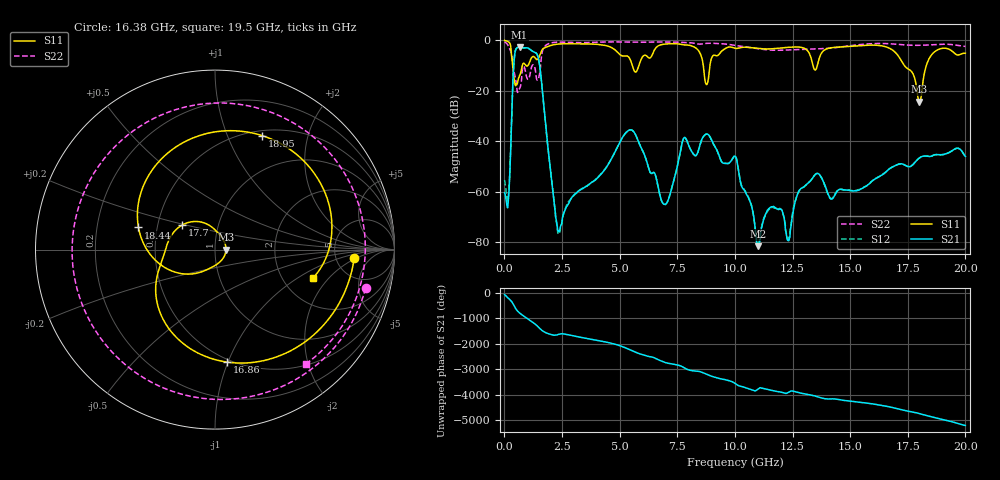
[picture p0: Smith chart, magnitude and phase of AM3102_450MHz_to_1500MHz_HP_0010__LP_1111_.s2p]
!Agilent Technologies,E8364B,MY43040894,A.07.50.67
!Agilent E8364B: A.07.50.67
!Date: Thursday, January 11, 2018 05:29:24
!Correction: S11(Full 2 Port(1,2))
!S21(Full 2 Port(1,2))
!S12(Full 2 Port(1,2))
!S22(Full 2 Port(1,2))
!S2P File: Measurements: S11, S21, S12, S22:
# Hz S  dB  R 50
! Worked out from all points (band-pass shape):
!   1601 points, 10 MHz to 20 GHz, reference 50 ohm
!   highest |S21| = -2.68 dB at 659.7 MHz (marker M1); lowest = -81.5 dB at 11.02 GHz (marker M2)
!   |S21| within 3 dB of the highest: 446.7 MHz to 1.425 GHz (978.7 MHz wide, 105 % of centre)
!   lowest |S11| = -24.3 dB at 18 GHz (marker M3), VSWR 1.13, Z = 56.5 + j0.022 ohm
!   |S11| at or under -10 dB: 357.9 MHz to 776.6 MHz (418.6 MHz wide, 73.8 % of centre); 5.551 GHz to 5.833 GHz (282 MHz wide, 4.95 % of centre); 17.35 GHz to 18.3 GHz (949.2 MHz wide, 5.32 % of centre)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
!   |S22| runs from -20.6 to -0.6 dB; largest |S21 - S12| = 0.0028
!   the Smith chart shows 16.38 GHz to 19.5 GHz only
!   S11 on the Smith chart (normalised r, x): 16.38 GHz: 7.50, -1.82; 16.86 GHz: 0.48, -0.99; 17.7 GHz: 0.67, +0.19; 18.44 GHz: 0.39, +0.12; 18.95 GHz: 0.56, +1.34; 19.5 GHz: 2.95, -1.37
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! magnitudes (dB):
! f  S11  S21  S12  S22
! 10 MHz  -0.1  -60.3  -55.3  -0.6
! 172.4 MHz  -0.6  -63.7  -61.7  -2.3
! 434.8 MHz  -16.1  -6.6  -6.6  -13.1
! 659.7 MHz  -14.1  -2.7  -2.7  -19.1
! 1.484 GHz  -7.0  -7.5  -7.5  -15.0
! 2.321 GHz  -1.5  -75.3  -76.3  -0.7
! 3.346 GHz  -1.4  -58.9  -58.7  -0.9
! 5.47 GHz  -7.8  -35.4  -35.4  -0.7
! 6.682 GHz  -2.2  -58.5  -58.6  -0.7
! 7.819 GHz  -1.8  -38.4  -38.4  -0.9
! 10.01 GHz  -3.1  -45.8  -45.8  -2.0
! 11.02 GHz  -3.2  -81.5  -80.2  -3.4
! 13.34 GHz  -8.2  -54.9  -54.9  -3.4
! 16.38 GHz  -2.2  -53.3  -53.2  -1.2
! 16.68 GHz  -3.0  -51.0  -51.1  -1.3
! 16.86 GHz  -4.0  -50.0  -50.0  -1.5
! 17.7 GHz  -12.8  -49.4  -49.3  -2.0
! 18 GHz  -24.3  -46.6  -46.6  -2.0
! 18.44 GHz  -7.1  -46.0  -46.0  -1.8
! 18.95 GHz  -3.3  -45.3  -45.3  -1.5
! 19.5 GHz  -4.9  -43.2  -43.2  -1.8
! 20 GHz  -5.1  -45.9  -46.1  -2.4
